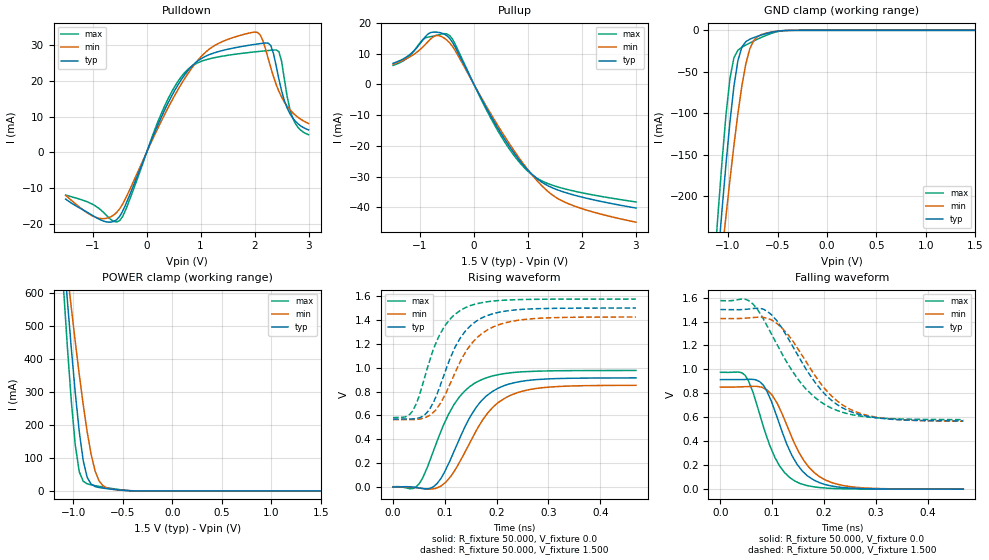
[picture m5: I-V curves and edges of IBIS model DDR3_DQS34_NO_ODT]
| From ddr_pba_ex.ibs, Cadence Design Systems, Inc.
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|   Model DDR3_DQS34_NO_ODT
[Model]   DDR3_DQS34_NO_ODT
Model_type I/O
Polarity   Non-Inverting
Enable   Active-High
Vinl   =   0.575V
Vinh   =   0.925V
C_comp   1.612pF   1.589pF   1.674pF
C_comp_pullup   0.458pF   0.493pF   0.466pF
C_comp_pulldown 1.154pF   1.097pF   1.207pF
[Model Spec]
Vinh   0.925V   NA   NA
Vinl   0.575V   NA   NA
Vmeas   0.750V   NA   NA
[Temperature Range]   27.000   0.125k   -40.000
[Voltage Range]   1.500V   1.425V   1.575V
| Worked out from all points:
|   slope of the pulldown table from 0 to 0.225 V, typ, clamps not added: 27.2 ohm
|   slope of the pullup table from 0 to 0.225 V, typ, clamps not added: 29.9 ohm
|   GND clamp passes 1 mA (typ) near -0.50 V on its own axis
|   POWER clamp passes 1 mA (typ) near -0.45 V on its own axis
|   rising waveform, R_fixture 50.000, V_fixture 0.0: 20-80 % time 66.9ps typ, 72.5ps min, 64.4ps max; typ from 0 V to 0.915 V
|   rising waveform, R_fixture 50.000, V_fixture 1.500: 20-80 % time 58.4ps typ, 66.4ps min, 52.7ps max; typ from 0.569 V to 1.5 V
|   falling waveform, R_fixture 50.000, V_fixture 0.0: 20-80 % time 53.8ps typ, 60.1ps min, 49ps max; typ from 0.915 V to 0 V
|   falling waveform, R_fixture 50.000, V_fixture 1.500: 20-80 % time 87.5ps typ, 87.7ps min, 90.3ps max; typ from 1.5 V to 0.57 V
[Pulldown]
|Voltage   I(typ)   I(min)   I(max)
-1.5V     -13.11mA   -12.09mA   -11.99mA
-900mV    -18.6mA    -18.43mA   -15.54mA
-500mV    -17.95mA   -15.85mA   -19.12mA
250mV     9.123mA    8.086mA    10.11mA
600mV     19.39mA    18.08mA    20.34mA
1.1V      27mA       28.19mA    25.96mA
1.7V      29.51mA    32.65mA    27.63mA
2.1V      30.49mA    33.01mA    28.32mA
2.3V      29.93mA    23.73mA    28.62mA
2.45V     20.53mA    17.11mA    28.23mA
2.7V      9.751mA    11.19mA    9.851mA
3V        6.277mA    8.093mA    4.942mA
[Pullup]
|Voltage   I(typ)   I(min)   I(max)
-1.5V     6.892mA    6.626mA    6.196mA
-1.2V     9.586mA    8.882mA    9.221mA
-950mV    14.51mA    12.17mA    14.57mA
-800mV    16.94mA    14.89mA    15.59mA
-650mV    16.95mA    15.91mA    16.25mA
-500mV    15.86mA    14.42mA    16.44mA
-350mV    12.21mA    11.08mA    13.19mA
450mV     -14.47mA   -13.63mA   -15.32mA
1V        -27.96mA   -27.83mA   -28.29mA
1.35V     -32.83mA   -34.57mA   -32.17mA
1.65V     -34.98mA   -38.1mA    -33.88mA
3V        -40.28mA   -44.89mA   -38.3mA
[GND_clamp]
|Voltage   I(typ)   I(min)   I(max)
-1.5V     -902.4mA   -795.2mA   -923mA
-1.14V    -333.6mA   -361.2mA   -285.4mA
-1.1V     -273.5mA   -314.1mA   -219.4mA
-1.06V    -215.4mA   -267.9mA   -157.1mA
-1.02V    -160.2mA   -222.9mA   -101.2mA
-980mV    -109.7mA   -179.4mA   -57.37mA
-940mV    -66.97mA   -138.2mA   -32.78mA
-900mV    -36.37mA   -100.2mA   -23.99mA
-820mV    -13.67mA   -40.29mA   -17.69mA
-740mV    -8.766mA   -12.21mA   -12.83mA
-540mV    -1.803mA   -1.643mA   -2.86mA
1.5V      1.904nA    275.5nA    464.3pA
[POWER_clamp]
|Voltage   I(typ)   I(min)   I(max)
-1.5V     2.395A     1.917A     2.689A
-1.1V     728.2mA    767.9mA    617.4mA
-1.06V    575.5mA    659.2mA    435.4mA
-1.02V    430.1mA    553.1mA    270.8mA
-980mV    295.8mA    450.4mA    137.9mA
-940mV    179.3mA    352.3mA    58.02mA
-900mV    91.53mA    260.8mA    29.3mA
-860mV    41.11mA    178.7mA    21.47mA
-780mV    13.3mA     60.49mA    15.94mA
-740mV    10.3mA     30.45mA    13.76mA
-620mV    5.486mA    5.676mA    7.71mA
1.5V      -5.523nA   -199nA     -1.165nA
[Ramp]
| variable   typ   min   max
dV/dt_r 0.549/67.274p   0.512/74.383p   0.586/65.956p
dV/dt_f 0.559/88.706p   0.516/90.109p   0.597/91.626p
R_load = 50.000
| The next line is not an IBIS keyword
| [Initial Delay]   0.225ns   0.350ns   0.175ns
[Rising Waveform]
R_fixture= 50.000
V_fixture= 0.0
V_fixture_min= 0.0
V_fixture_max= 0.0
|time   V(typ)   V(min)   V(max)
0s        454.9uV    1.58mV     3.018mV
45ps      -3.51mV    -5.637mV   3.089mV
57ps      -12.27mV   -12.07mV   74.62mV
85ps      29.19mV    -6.197mV   383.8mV
102ps     148.8mV    41.77mV    562mV
126ps     381.7mV    189.6mV    743.7mV
171ps     723.9mV    548.6mV    899.9mV
203ps     828.2mV    708.2mV    941.9mV
258ps     892.2mV    812.2mV    967.5mV
469ps     914.6mV    852.4mV    976.8mV
[Rising Waveform]
R_fixture= 50.000
V_fixture= 1.500
V_fixture_min= 1.425
V_fixture_max= 1.575
|time   V(typ)   V(min)   V(max)
0s        569.3mV    565.6mV    582mV
38ps      571mV      564.5mV    638.1mV
51ps      580.6mV    569.3mV    770mV
69ps      641.2mV    596.6mV    1.035V
99ps      947.3mV    761.1mV    1.344V
119ps     1.166V     950.8mV    1.445V
139ps     1.304V     1.124V     1.502V
172ps     1.418V     1.288V     1.545V
228ps     1.481V     1.387V     1.568V
469ps     1.5V       1.425V     1.575V
[Falling Waveform]
R_fixture= 50.000
V_fixture= 0.0
V_fixture_min= 0.0
V_fixture_max= 0.0
|time   V(typ)   V(min)   V(max)
0s        914.8mV    852.4mV    976.1mV
48ps      916.2mV    856.6mV    948.7mV
62ps      916.6mV    859.3mV    822mV
83ps      867.7mV    844.5mV    522.2mV
100ps     716.4mV    784.3mV    316.6mV
114ps     543.6mV    679.1mV    195.9mV
145ps     230.1mV    365.4mV    65.5mV
180ps     77.6mV     142.5mV    19.75mV
225ps     19.34mV    42.2mV     4.648mV
469ps     168.9uV    121.2uV    85.85uV
[Falling Waveform]
R_fixture= 50.000
V_fixture= 1.500
V_fixture_min= 1.425
V_fixture_max= 1.575
|time   V(typ)   V(min)   V(max)
0s        1.5V       1.424V     1.574V
54ps      1.504V     1.43V      1.576V
71ps      1.511V     1.435V     1.505V
98ps      1.459V     1.414V     1.3V
129ps     1.273V     1.299V     1.055V
155ps     1.076V     1.136V     888.4mV
213ps     747mV      785.6mV    679.6mV
246ps     657.4mV    677.1mV    629.7mV
295ps     600.2mV    605.8mV    597.9mV
469ps     570mV      567.1mV    580.7mV
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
